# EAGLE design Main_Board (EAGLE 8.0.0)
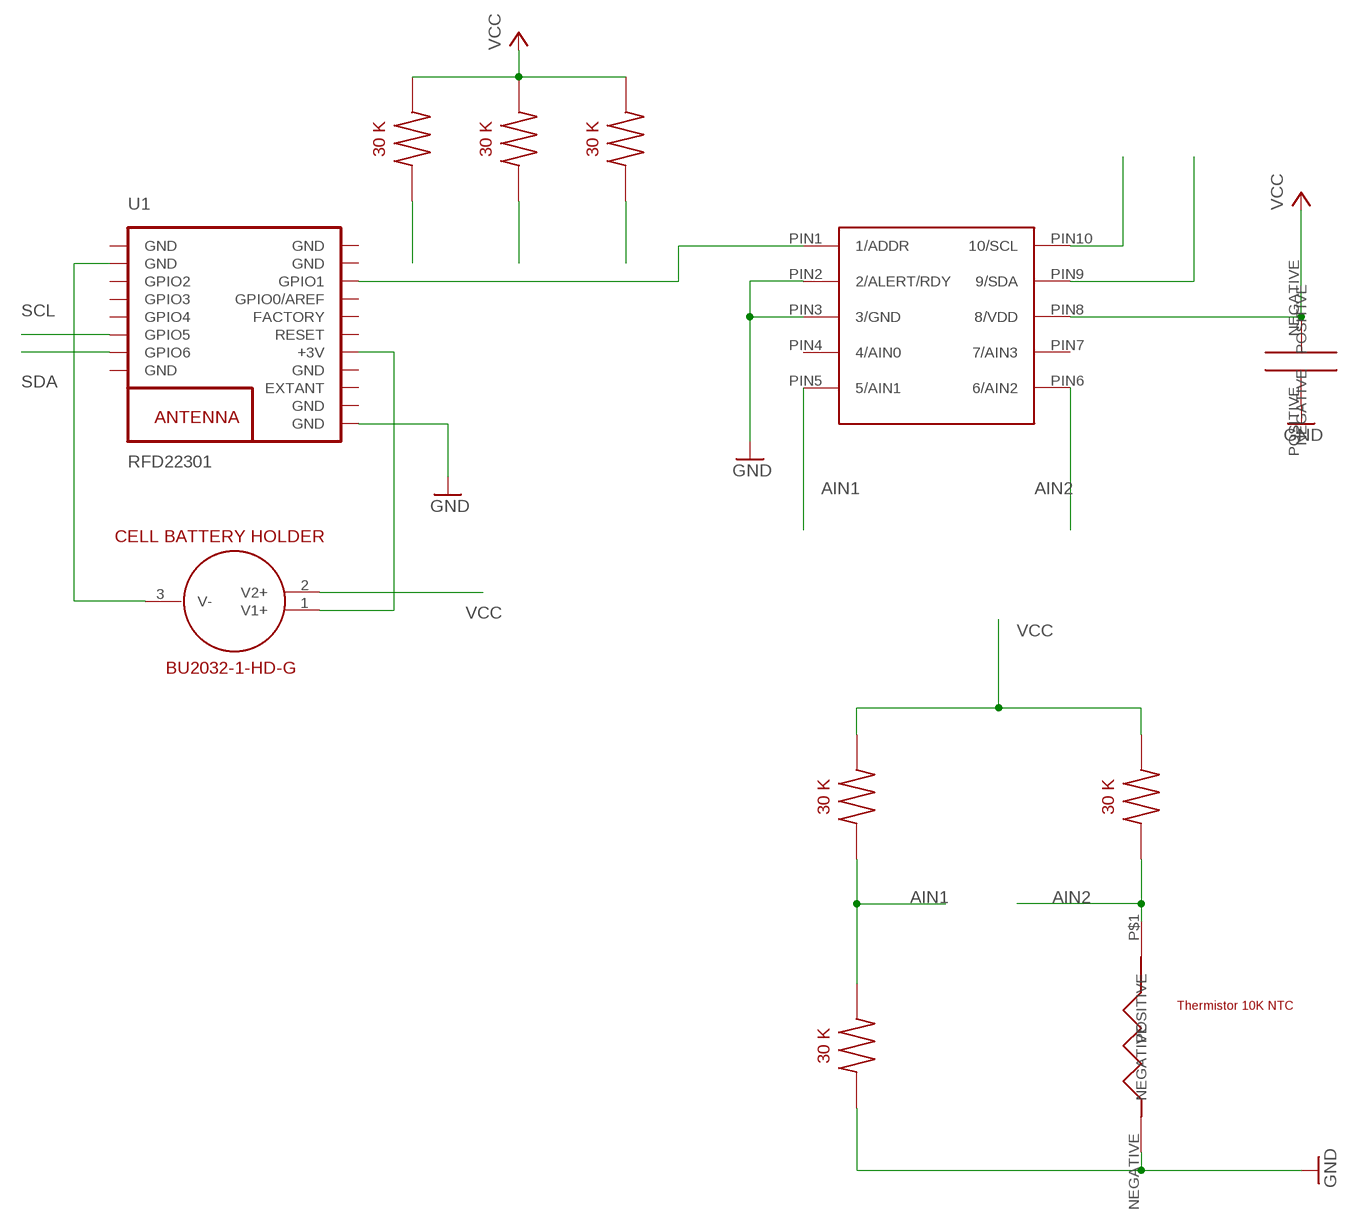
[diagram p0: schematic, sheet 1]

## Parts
U1  RFD22301  [RFD22301]
U$1  ADS1115_DGS  [ADS1115_DGS]
U$2  THERMISTOR_NTC_10K  [THERMISTOR_NTC_10K]
U$3  30K_TH_RESISTOR_1135-1507  [1135-1507]
U$4  30K_TH_RESISTOR_1135-1507  [1135-1507]
U$5  30K_TH_RESISTOR_1135-1507  [1135-1507]
U$7  BATTERY_HOLDER_BU2032-1-HD-G  [BU2032-1-HD-G]
U$11  30K_TH_RESISTOR_1135-1507  [1135-1507]
U$12  30K_TH_RESISTOR_1135-1507  [1135-1507]
U$13  30K_TH_RESISTOR_1135-1507  [1135-1507]
U$14  CERAM_CAP_0.1UF  [CAP_CERAMIC_0.1UF]

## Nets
AIN1: U$1.PIN5(5/AIN1) U$4.1 U$5.2
AIN2: U$1.PIN6(6/AIN2) U$2.P$1(POSITIVE) U$3.1
GND: U1.9(GND) U$1.PIN2(2/ALERT/RDY) U$1.PIN3(3/GND) U$2.NEGATIVE U$5.1 U$14.POSITIVE
N$2: U1.2(GND) U$7.3(V-)
N$3: U1.17(GPIO1) U$1.PIN1(1/ADDR)
POWER_BUS: U1.13(+3V) U$7.1(V1+)
SCL: U1.6(GPIO5) U$1.PIN10(10/SCL) U$11.1
SDA: U1.7(GPIO6) U$1.PIN9(9/SDA) U$12.1 U$13.1
VCC: U$1.PIN8(8/VDD) U$3.2 U$4.2 U$7.2(V2+) U$11.2 U$12.2 U$13.2 U$14.NEGATIVE
Unconnected: U1.3(GPIO2) U1.4(GPIO3) U1.5(GPIO4) U1.11(EXTANT) U1.14(RESET) U1.15(FACTORY) U1.16(GPIO0/AREF) U$1.PIN4(4/AIN0) U$1.PIN7(7/AIN3)

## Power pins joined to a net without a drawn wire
GND: U1.1(GND) U1.8(GND) U1.10(GND) U1.12(GND) U1.18(GND) U1.19(GND)

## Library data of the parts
U1 = RF_Digital_RFD22301_Eagle_Schematic_PCB_Library:RFD22301: RFD22301 RFduino SMT Module RFD22301 Datasheet: http://www.rfdigital.com/wp-content/uploads/2014/03/RFD22301.Data_.Sheet_.11.24.13_11.38PM.pdf
U$1 = ADS1115_DGS:ADS1115_DGS
U$2 = Thermistor_NTC_10K:THERMISTOR_NTC_10K
U$3-U$5 U$11-U$13 = QBiT_Em'sComponents:30K_TH_RESISTOR_1135-1507
U$7 = QBiT_Em'sComponents:BATTERY_HOLDER_BU2032-1-HD-G
U$14 = Cap_Ceram_0.1uf:CERAM_CAP_0.1UF

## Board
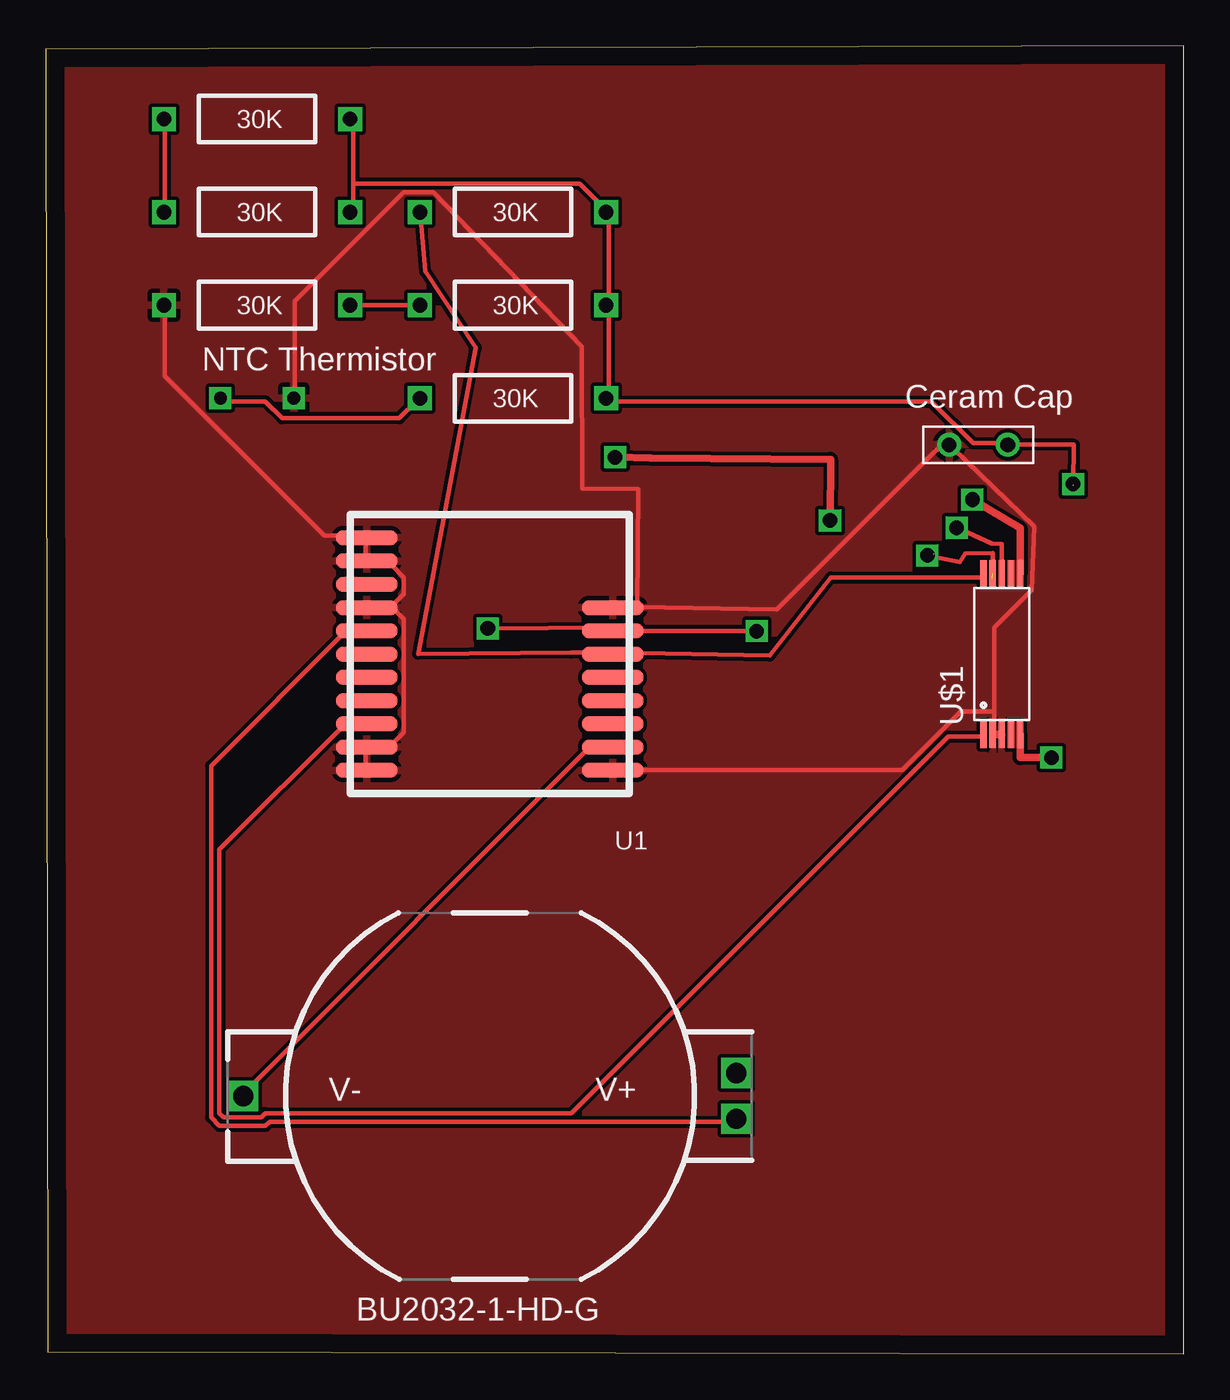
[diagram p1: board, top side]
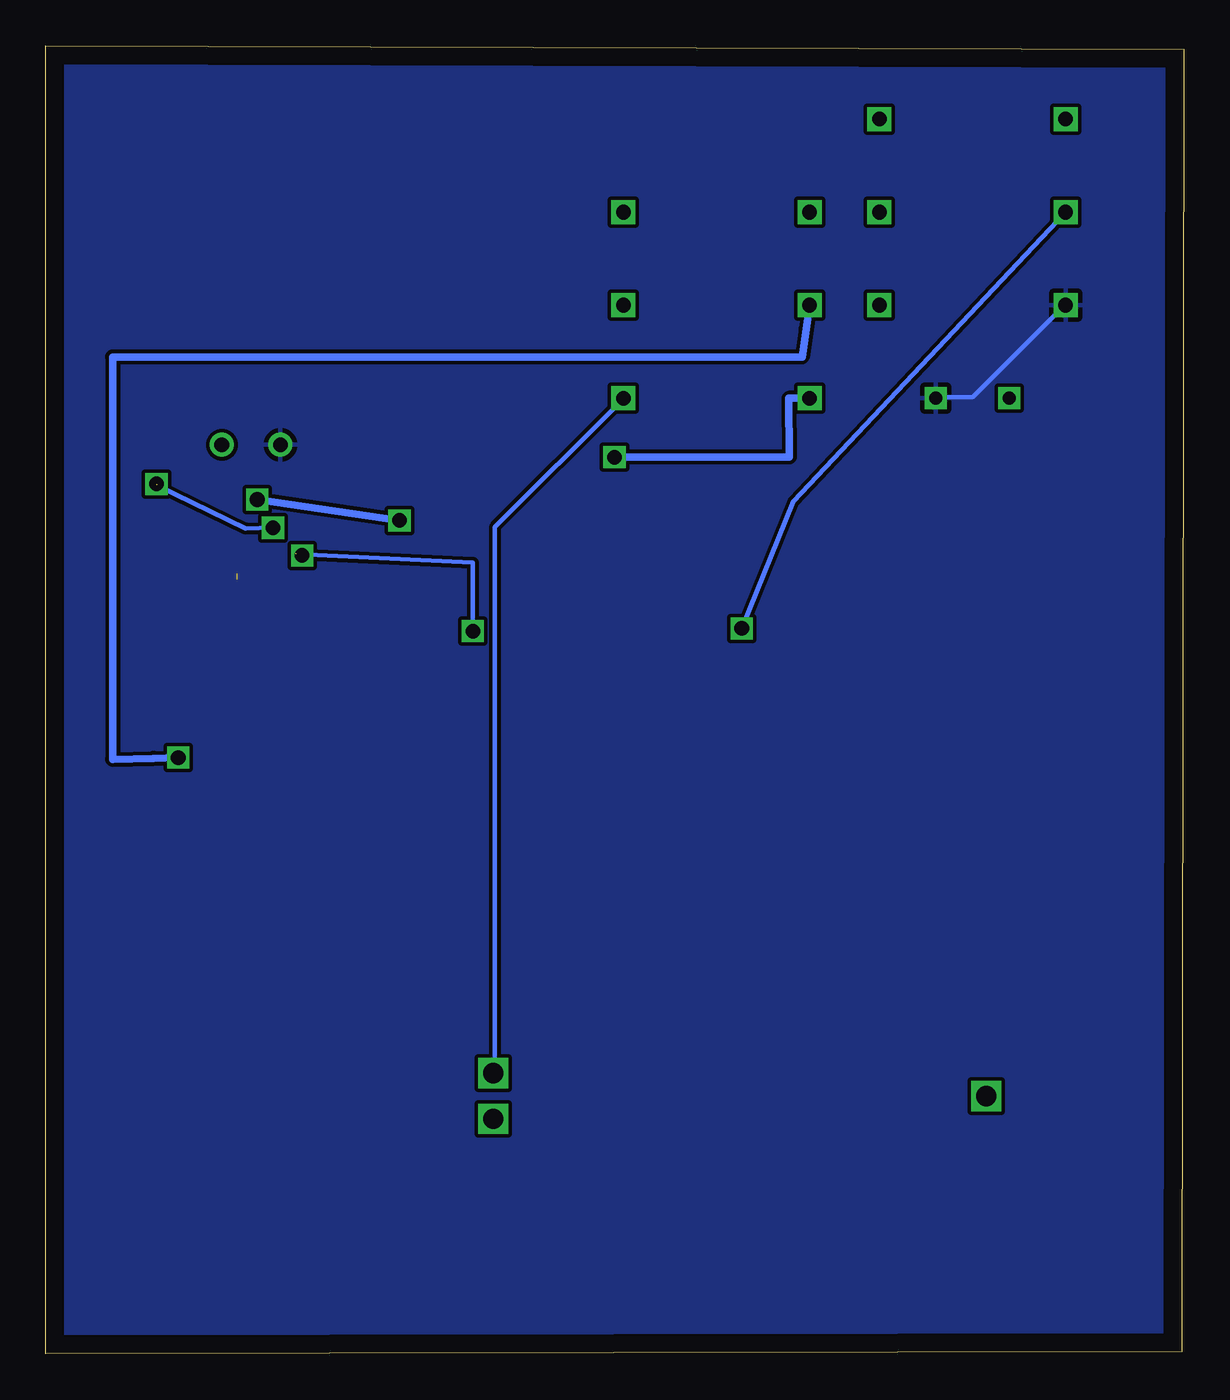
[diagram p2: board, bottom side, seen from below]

Size 62.11 x 71.41 mm. Coordinates in mm from the lower left corner, seen from the top.
Outline: 0.1,0.1 62.11,0 62.11,71.41 0,71.2 0.1,0.1
Copper layers (1*16): Top 0.035mm / dielectric 1.5mm / Bottom 0.035mm
Design rules "default": minimum track width 10mil, minimum drill 24mil, track to track 8mil, track to pad 8mil, pad to pad 8mil, via to via 8mil, smd to smd 8mil, copper to edge 40mil, drill to drill 8mil, minimum pad ring 10mil, minimum via ring 8mil, stop-mask expansion 4mil, vias tented up to drill 0mil, thermal gap 10mil

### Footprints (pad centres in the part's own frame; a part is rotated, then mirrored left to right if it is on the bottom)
RFD22301 = smd 3.353 x 0.813: 1 -6.706,7.62; 2 -6.706,6.35; 3 -6.706,5.08; 4 -6.706,3.81; 5 -6.706,2.54; 6 -6.706,1.27; 7 -6.706,0; 8 -6.706,-1.27; 9 6.706,-5.08; 10 6.706,-3.81; 11 6.706,-2.54; 12 6.706,-1.27; 13 6.706,0; 14 6.706,1.27; 15 6.706,2.54; 16 6.706,3.81; 17 6.706,5.08; 18 6.706,6.35; 19 6.706,7.62
ADS1115_DGS = smd 1.45 x 0.35: PIN1 -4.4,1; PIN2 -4.4,0.5; PIN3 -4.4,0; PIN4 -4.4,-0.5; PIN5 -4.4,-1; PIN6 4.4,-1; PIN7 4.4,-0.5; PIN8 4.4,0; PIN9 4.4,0.5; PIN10 4.4,1
THERMISTOR_NTC_10K = drill 0.7 square: NEGATIVE 2,0; P$1 -2,0
1135-1507 = drill 0.8 square: 1 -5.08,0; 2 5.08,0
BU2032-1-HD-G = drill 1.1 square: 1 -13.45,1.25; 2 -13.45,-1.25; 3 13.45,0
CAP_CERAMIC_0.1UF = drill 0.8 pad 1.25: NEGATIVE 1.6,0; POSITIVE -1.6,0

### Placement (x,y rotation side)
U1  24.23,39.46 180 top
U$1  52.17,38.2 90 top
U$2  11.53,52.16 0 top
U$3  25.5,52.16 0 top
U$4  25.5,57.24 0 top
U$5  11.53,57.24 0 top
U$7  24.23,14.07 180 top
U$11  25.5,62.32 0 top
U$12  11.53,62.32 0 top
U$13  11.53,67.41 0 top
U$14  50.9,49.62 0 top

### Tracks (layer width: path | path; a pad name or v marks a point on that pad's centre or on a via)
AIN1  (via drill 0.8)
  Top 0.254: U$5.2 U$4.1
  Top 0.406: v54.88,32.55 53.17,32.55 U$1.PIN5
  Bottom 0.406: U$4.1 20.62,55.94 20.84,54.42 58.45,54.42 58.45,32.45 56.23,32.5 v54.88,32.55
AIN2  (via drill 0.8)
  Top 0.254: U$2.P$1 9.7,51.99 11.99,51.99 12.9,51.07 19.3,51.07 20.22,51.99 U$3.1
  Top 0.406: v31.07,48.95 33.02,48.89 42.83,48.82 v42.8,45.49 | v50.57,46.63 53.17,45.07 U$1.PIN6
  Bottom 0.406: U$3.1 21.55,52.16 21.53,48.95 v31.07,48.95 | v42.8,45.49 v50.57,46.63
GND
  Top 0.254: U1.19 17.47,31.87 17.47,33.01 U1.18 17.7,33.24 18.85,33.24 19.53,33.93 19.53,40.1 18.85,40.79 | 18.85,40.79 17.7,40.79 U1.12 18.85,40.79 | 18.85,40.79 19.53,41.47 19.53,42.39 18.85,43.07 17.7,43.07 U1.10 17.47,43.3 17.47,44.44 U1.9 17.47,44.67 15.19,44.67 6.5,53.36 6.5,57.24 U$5.1 | 51.76,35.07 51.76,39.64 53.82,41.7 53.96,45.15 49.48,49.47 U$14.POSITIVE 48.58,49.33 39.9,40.64 32.28,40.76 | 51.76,35.07 51.76,33.93 U$1.PIN2 | 51.76,35.07 49.94,35.07 46.73,31.87 30.96,31.87 U1.1 | 32.28,40.76 32.31,40.76 30.96,40.79 U1.8 30.73,40.79 | U$2.NEGATIVE 13.59,52.22 13.59,57.47 19.53,63.42 21.13,63.42 29.25,54.98 29.27,47.23 32.34,47.2 | 32.33,47.19 32.28,40.76
  Top 0.406: U$1.PIN2 U$1.PIN3
  Bottom 0.254: U$2.NEGATIVE 13.36,52.22 11.53,52.22 6.5,57.24 U$5.1
  pour Bottom (isolate 0.012): 0.23,71.11 0.3,0.3 61.98,0.3 61.98,0.49 61.88,0.49 61.88,71.14
  pour Top: 0.24,70.62 0.35,0.56 58.19,0.68 61.35,0.66 61.35,70.91 0.38,70.91
N$2
  Top 0.254: U$7.3 10.84,14.27 29.59,33.01 30.73,33.01 U1.2
N$3
  Top 0.254: U1.17 16.33,34.38 9.47,27.53 9.47,13.12 9.7,12.9 11.76,12.9 11.99,13.12 28.68,13.12 49.25,33.7 51.08,33.7 U$1.PIN1
POWER_BUS
  Top 0.254: U$7.1 37.59,12.67 12.22,12.67 11.99,12.44 9.47,12.44 9.01,12.9 9.01,32.1 16.33,39.41 17.47,39.41 U1.13
SCL
  Top 0.254: U$1.PIN10 51.08,42.39 42.85,42.39 39.5,38.11 30.96,38.27 U1.6 30.73,38.27 28.68,38.27 20.32,38.21 23.47,54.91 20.7,59.1 20.45,62.27 U$11.1
SDA  (via drill 0.8)  (2 unrouted)
  Top 0.254: U$12.1 6.5,62.5 6.5,67.3 U$13.1 | v24.12,39.6 30.73,39.64 U1.7 38.5,39.46 | 48.49,43.69 v48.12,43.59 49.88,43.22 50.18,43.68 51.68,43.7 51.69,43.41 51.66,42.3
  Top 0.406: 38.5,39.46 v38.8,39.45
  Bottom 0.254: v24.12,39.6 21.3,46.53 U$12.1 | 48.43,43.66 38.8,43.19 v38.8,39.45
VCC  (via drill 0.8)  (1 unrouted)
  Top 0.254: 16.79,63.87 16.79,67.3 U$13.2 | 16.79,63.87 16.79,62.5 U$12.2 | 30.73,57.24 30.73,52.22 U$3.2 30.73,51.99 48.34,51.99 50.62,49.7 52.45,49.7 U$14.NEGATIVE 56.11,49.62 v56.07,47.48 | 30.73,57.24 30.73,62.27 U$11.2 30.5,62.5 29.13,63.87 16.79,63.87 | 30.73,57.24 U$4.2 | 56.08,47.47 56.05,47.45 | v49.7,45.09 51.58,44.24 51.62,44.23 52.17,44.21 U$1.PIN8
  Top 0.406: v56.07,47.48 56.08,47.47
  Bottom 0.254: U$7.2 37.59,15.41 37.59,45.13 30.73,51.99 U$3.2 | 56.07,47.41 51.18,45.05 51.23,45.05 v49.7,45.09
